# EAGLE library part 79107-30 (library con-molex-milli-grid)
RECEPTACAL
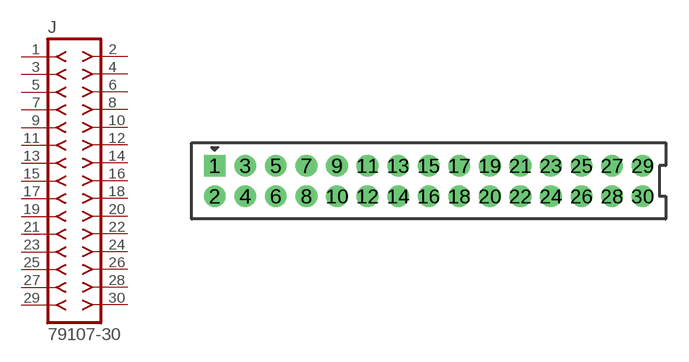
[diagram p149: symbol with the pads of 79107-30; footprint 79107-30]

Designator prefix J

## 79107-30  [79107-30]
1  1  pas
2  2  pas
3  3  pas
4  4  pas
5  5  pas
6  6  pas
7  7  pas
8  8  pas
9  9  pas
10  10  pas
11  11  pas
12  12  pas
13  13  pas
14  14  pas
15  15  pas
16  16  pas
17  17  pas
18  18  pas
19  19  pas
20  20  pas
21  21  pas
22  22  pas
23  23  pas
24  24  pas
25  25  pas
26  26  pas
27  27  pas
28  28  pas
29  29  pas
30  30  pas

## Footprint 79107-30 (pad centres in mm)
RECEPTACAL Dual Row, Vertical, Through-Hole
drill 0.914 square: 1 -14,1
drill 0.914: 2 -14,-1; 3 -12,1; 4 -12,-1; 5 -10,1; 6 -10,-1; 7 -8,1; 8 -8,-1; 9 -6,1; 10 -6,-1; 11 -4,1; 12 -4,-1; 13 -2,1; 14 -2,-1; 15 0,1; 16 0,-1; 17 2,1; 18 2,-1; 19 4,1; 20 4,-1; 21 6,1; 22 6,-1; 23 8,1; 24 8,-1; 25 10,1; 26 10,-1; 27 12,1; 28 12,-1; 29 14,1; 30 14,-1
